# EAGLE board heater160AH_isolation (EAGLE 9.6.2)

Size 280 x 92 mm. Coordinates in mm from the lower left corner, seen from the top.
Outline: 0,0 0,92 125,92 125,82 155,82 155,92 280,92 280,0 0,0
Copper layers (1*16): Top 0.035mm / dielectric 1.5mm / Bottom 0.035mm
Design rules "default": minimum track width 6mil, minimum drill 0.35mm, track to track 6mil, track to pad 6mil, pad to pad 6mil, via to via 6mil, smd to smd 6mil, copper to edge 40mil, drill to drill 6mil, minimum pad ring 10mil, minimum via ring 8mil, stop-mask expansion 4mil, vias tented up to drill 0mil, thermal gap 10mil

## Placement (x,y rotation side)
U$1  [CE-4MM]  54.04,76.14 0 top

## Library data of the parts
U$1 = logo

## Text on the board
tPlace: ECS, Am Wenigerflur 14, 54498 Piesport | HEATER280_304 | ISOLATION PLATE / (END PLATE)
